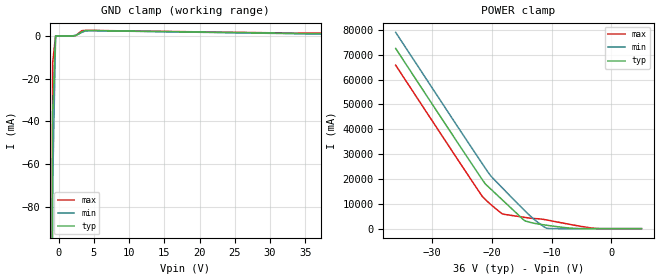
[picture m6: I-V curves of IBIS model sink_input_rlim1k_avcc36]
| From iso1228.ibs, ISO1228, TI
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|   Model sink_input_rlim1k_avcc36
[Model] sink_input_rlim1k_avcc36
Model_type Input
Vinl =  5.100V
Vinh =  6.000V
C_comp   0.859pF   0.874pF   1.06pF
[Model Spec]
Vinh   6.000V   5.700V   6.400V
Vinl   5.100V   4.700V   5.300V
[Temperature Range]   27.000   150   -40
[Voltage Range]   36.000V   36.000V   36.000V
[GND_clamp]
|Voltage   I(typ)   I(min)   I(max)
-36V      -59.67A    -59.3A     -59.9A
-1.273V   -477.6mA   -508mA     -473.9mA
-859mV    -36.12mA   -70.17mA   -12.47mA
-444mV    -570nA     -59.15uA   -630nA
2.04V     18.94uA    92.16uA    12.24uA
2.455V    216.4uA    384.5uA    222.5uA
3.283V    2.001mA    1.638mA    2.443mA
3.697V    2.442mA    2.229mA    2.561mA
4.939V    2.514mA    2.455mA    2.582mA
33.93V    1.169mA    1.019mA    1.312mA
72V       -541uA     -819.7uA   935.1uA
[POWER_clamp]
|Voltage   I(typ)   I(min)   I(max)
-36V      72.54A     79A        65.79A
-21.5V    19.55A     25.97A     12.83A
-21.09V   18.14A     24.49A     11.84A
-20.26V   16.22A     21.61A     9.992A
-18.19V   11.53A     16.36A     5.913A
-14.46V   3.172A     7.235A     4.531A
-12.39V   1.947A     2.745A     3.999A
-10.74V   1.347A     97.87mA    3.471A
-6.182V   90.39mA    49.82uA    1.383A
-2.869V   13.02uA    -218.9nA   153.8mA
5V        0A         0A         0A
